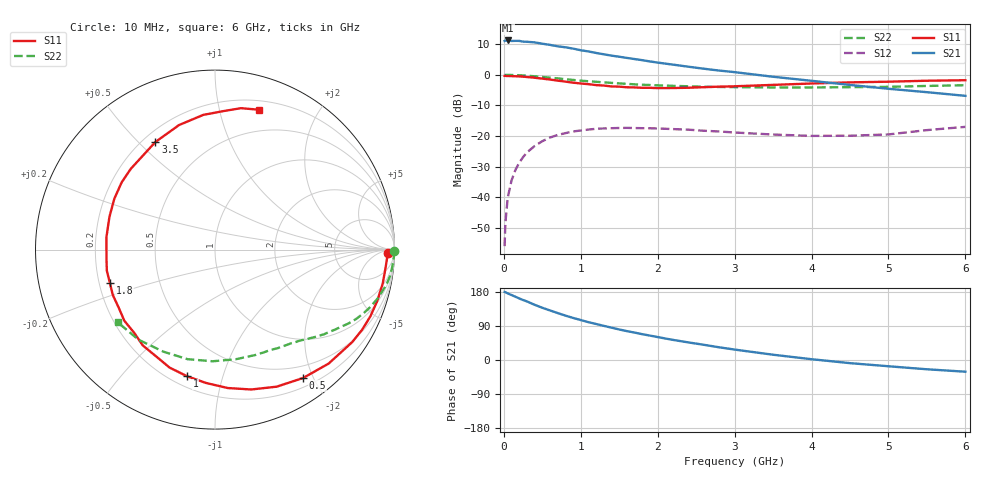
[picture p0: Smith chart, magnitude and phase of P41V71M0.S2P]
! SIEMENS Small Signal Semiconductors
! BFP182
! Si NPN RF Bipolar Junction Transistor in SOT143
! VCE = 1.75 V  IC = 1 mA
! Common Emitter S-Parameters:  March  1996
# GHz  S  MA  R  50
!  f  S11  S21  S12  S22
! GHz  MAG  ANG  MAG  ANG  MAG  ANG  MAG  ANG
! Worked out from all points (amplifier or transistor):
!   36 points, 10 MHz to 6 GHz, reference 50 ohm
!   highest |S21| = 11.2 dB at 50 MHz (marker M1)
!   |S21| within 3 dB of that: start of sweep to 964 MHz
!   unconditionally stable (mu >= 1): 2.586 GHz to end of sweep
!   at 250 MHz: K = 0.10, MSG = 18.8 dB, |S12| = -26.9 dB
!   at 1.4 GHz: K = 0.54, MSG = 11.8 dB, |S12| = -17.4 dB
!   at 6 GHz: K = 1.10, MAG = 3.1 dB, |S12| = -17.0 dB
!   S11 on the Smith chart (normalised r, x): 10 MHz: 41, -20; 500 MHz: 0.32, -1.85; 1 GHz: 0.26, -0.77; 1.8 GHz: 0.24, -0.14; 3.5 GHz: 0.25, +0.56; 6 GHz: 0.28, +1.32
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0.01  0.9613 -1.1  3.566 179.5  0.0016 85.6  0.9981 -0.4
0.02  0.9607 -2.3  3.603 179.0  0.0038 85.3  0.997 -0.8
0.05  0.9562 -5.6  3.638 175.8  0.0098 85.8  0.9975 -2.2
0.1  0.9535 -11.4  3.568 171.4  0.0189 82.3  0.9937 -4.4
0.2  0.9423 -23.2  3.578 162.5  0.0368 75.5  0.9856 -8.7
0.4  0.8967 -45.1  3.386 145.7  0.0689 62.2  0.9468 -16.6
0.5  0.8674 -55.6  3.219 137.8  0.0827 55.9  0.923 -20.2
0.6  0.8374 -65.8  3.082 130.8  0.0946 50.3  0.8998 -23.3
0.8  0.7746 -84.7  2.815 117.2  0.1118 40.1  0.8495 -29.0
0.9  0.7446 -93.9  2.679 111.1  0.1191 35.6  0.8254 -31.3
1  0.7224 -102.5  2.519 105.4  0.1234 31.4  0.8036 -33.7
1.1  0.7043 -111.1  2.407 99.8  0.1279 27.6  0.7852 -35.7
1.3  0.6685 -127.0  2.162 90.1  0.1334 20.7  0.7534 -39.5
1.5  0.6421 -141.9  1.975 80.6  0.1357 15.1  0.724 -43.0
1.8  0.6142 -162.5  1.734 68.1  0.1347 8.9  0.6898 -47.6
2.2  0.6089 173.5  1.466 53.0  0.1302 1.8  0.6607 -54.2
2.8  0.6411 144.1  1.173 33.5  0.119 -3.9  0.6337 -64.7
3.5  0.6854 119.0  0.93 13.9  0.1061 -4.0  0.6218 -79.3
4  0.7223 106.1  0.799 2.1  0.1008 0.1  0.6223 -91.2
4.5  0.7533 95.0  0.684 -8.3  0.1014 4.7  0.6293 -104.0
5.5  0.8011 79.6  0.521 -24.5  0.1253 14.1  0.6586 -130.3
6  0.8166 72.7  0.454 -30.9  0.1416 13.2  0.6767 -143.2
